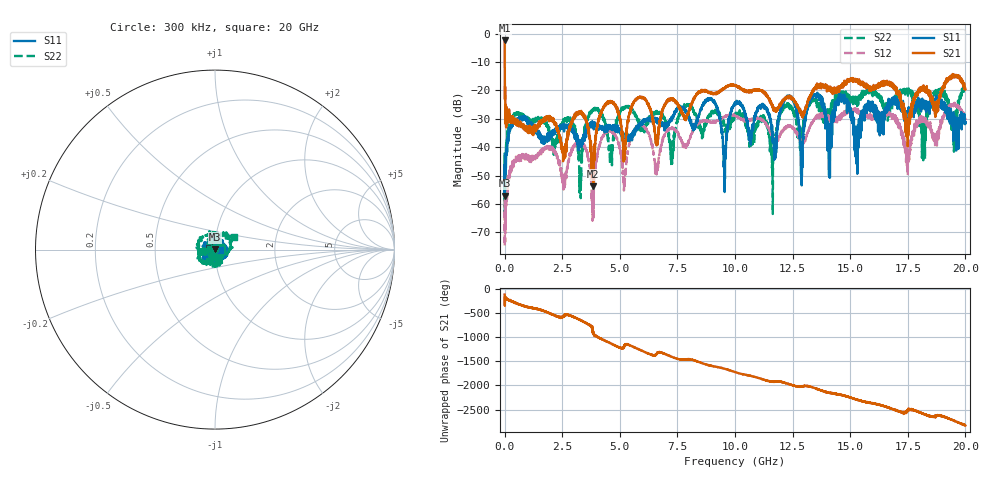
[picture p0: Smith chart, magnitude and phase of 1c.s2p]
!Keysight Technologies,N5232A,MY52221221,A.10.65.11
!Date: Thursday, August 21, 2025 19:55:20
!Correction: S11(Full 2 Port(1,4))
!S41(Full 2 Port(1,4))
!S14(Full 2 Port(1,4))
!S44(Full 2 Port(1,4))
!S2P File: Measurements: S11, S41, S14, S44:
# Hz S  RI  R 50
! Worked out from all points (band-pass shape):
!   4001 points, 300 kHz to 20 GHz, reference 50 ohm
!   highest |S21| = -2.39 dB at 300 kHz (marker M1); lowest = -53.7 dB at 3.845 GHz (marker M2)
!   |S21| within 3 dB of the highest: start of sweep to 1.903 MHz
!   lowest |S11| = -57.0 dB at 5.3 MHz (marker M3), VSWR 1.00, Z = 50 + j0.14 ohm
!   |S11| at or under -10 dB: start of sweep to end of sweep
!   |S22| runs from -63.5 to -17.8 dB; largest |S21 - S12| = 0.76
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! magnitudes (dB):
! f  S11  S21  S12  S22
! 300 kHz  -42.3  -2.4  -53.9  -42.7
! 5.3 MHz  -57.0  -11.8  -74.8  -62.8
! 160.3 MHz  -35.6  -30.0  -51.6  -34.8
! 2.555 GHz  -33.0  -43.8  -54.9  -30.3
! 3.335 GHz  -38.5  -28.3  -38.7  -42.4
! 3.845 GHz  -31.8  -53.7  -58.0  -26.5
! 4.5 GHz  -33.4  -24.2  -34.4  -37.5
! 6.67 GHz  -30.5  -34.5  -44.7  -28.2
! 8.995 GHz  -23.1  -21.2  -31.3  -27.6
! 9.555 GHz  -49.2  -19.0  -29.1  -32.5
! 10 GHz  -24.2  -18.2  -28.9  -28.2
! 11.65 GHz  -35.3  -25.8  -36.4  -46.8
! 12.42 GHz  -22.1  -22.4  -32.6  -25.3
! 12.91 GHz  -50.0  -28.0  -38.6  -37.2
! 13.34 GHz  -22.5  -20.9  -31.5  -23.5
! 14.09 GHz  -40.9  -20.1  -30.2  -26.6
! 14.6 GHz  -23.0  -18.8  -29.6  -21.2
! 15.27 GHz  -37.4  -16.6  -27.6  -23.5
! 16.67 GHz  -25.7  -17.6  -27.4  -28.3
! 17.49 GHz  -29.5  -32.6  -45.6  -19.8
! 18.19 GHz  -25.7  -18.6  -29.9  -36.8
! 20 GHz  -31.1  -19.6  -30.5  -18.0
